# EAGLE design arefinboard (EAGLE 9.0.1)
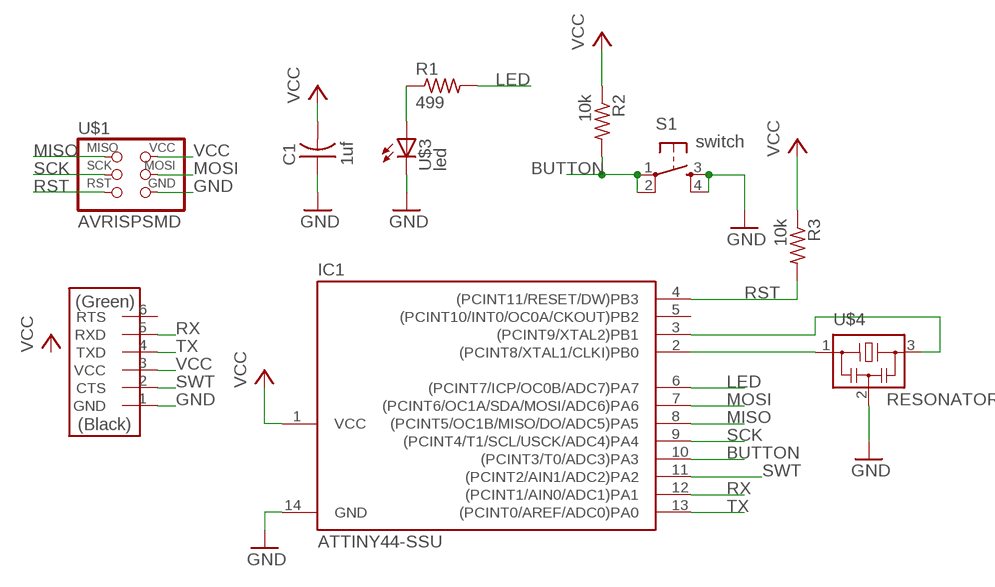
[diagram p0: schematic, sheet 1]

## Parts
C1  1uf  CAP-US1206FAB  [C1206FAB]
IC1  ATTINY44-SSU  [SOIC14]
R1  499  RES-US1206FAB  [R1206FAB]
R2  10k  RES-US1206FAB  [R1206FAB]
R3  10k  RES-US1206FAB  [R1206FAB]
S1  switch  6MM_SWITCH6MM_SWITCH  [6MM_SWITCH]
U$1  AVRISPSMD  [2X03SMD]
U$2  FTDI-SMD-HEADER  [1X06SMD]
U$3  led  LEDFAB1206  [LED1206FAB]
U$4  RESONATOR  [EFOBM]

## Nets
BUTTON: IC1.10((PCINT3/T0/ADC3)PA3) R2.2 S1.1(P) S1.2(P1)
GND: C1.1 IC1.14(GND) S1.3(S) S1.4(S1) U$1.6(GND) U$2.1(GND) U$3.2(C) U$4.2
LED: IC1.6((PCINT7/ICP/OC0B/ADC7)PA7) R1.2
MISO: IC1.8((PCINT5/OC1B/MISO/DO/ADC5)PA5) U$1.1(MISO)
MOSI: IC1.7((PCINT6/OC1A/SDA/MOSI/ADC6)PA6) U$1.4(MOSI)
N$1: R1.1 U$3.1(A)
N$10: IC1.3((PCINT9/XTAL2)PB1) U$4.3
N$11: IC1.2((PCINT8/XTAL1/CLKI)PB0) U$4.1
RST: IC1.4((PCINT11/RESET/DW)PB3) R3.2 U$1.5(RST)
RX: IC1.12((PCINT1/AIN0/ADC1)PA1) U$2.5(RXD)
SCK: IC1.9((PCINT4/T1/SCL/USCK/ADC4)PA4) U$1.3(SCK)
SWT: IC1.11((PCINT2/AIN1/ADC2)PA2) U$2.2(CTS)
TX: IC1.13((PCINT0/AREF/ADC0)PA0) U$2.4(TXD)
VCC: C1.2 IC1.1(VCC) R2.1 R3.1 U$1.2(VCC) U$2.3(VCC)
Unconnected: IC1.5((PCINT10/INT0/OC0A/CKOUT)PB2) U$2.6(RTS)

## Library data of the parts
C1 = fab:CAP-US
IC1 = fab:ATTINY44
R1-R3 = fab:RES-US: Resistor (US Symbol)
S1 = FabLab:6MM_SWITCH: OMRON SWITCH
U$1 = fab:AVRISP
U$2 = fab:FTDI-SMD-HEADER
U$3 = fab:LED: LED
U$4 = fab:RESONATOR

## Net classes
0 default: width 0.305 mm, drill 0.508 mm, clearance 0.254 mm

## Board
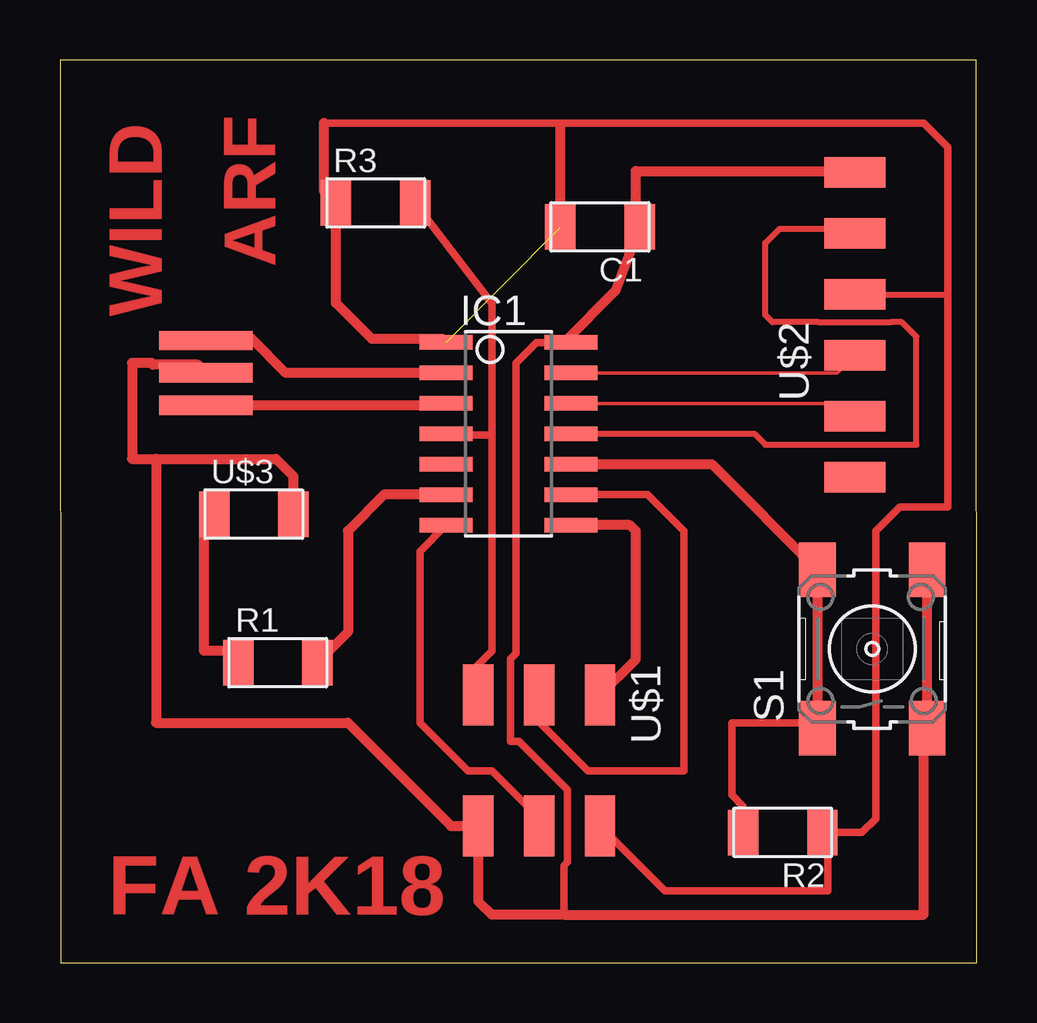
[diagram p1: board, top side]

Size 38.22 x 37.63 mm. Coordinates in mm from the lower left corner, seen from the top.
Outline: 0.03,0 38.22,0 38.19,37.63 0,37.63 0.03,0
Copper layers (1*16): Top 0.035mm / dielectric 1.5mm / Bottom 0.035mm
Design rules "default *": minimum track width 10mm, minimum drill 0.35mm, track to track 16mil, track to pad 16mil, pad to pad 16mil, via to via 16mil, smd to smd 16mil, copper to edge 40mil, drill to drill 6mil, minimum pad ring 10mil, minimum via ring 8mil, stop-mask expansion 4mil, vias tented up to drill 0mil, thermal gap 10mil

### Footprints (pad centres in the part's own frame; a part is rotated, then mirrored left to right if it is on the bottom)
C1206FAB = smd 1.27 x 1.905: 1 -1.651,0; 2 1.651,0
SOIC14 = smd 0.61 x 2.21: 1 -3.81,-2.603; 2 -2.54,-2.603; 3 -1.27,-2.603; 4 0,-2.603; 5 1.27,-2.603; 6 2.54,-2.603; 7 3.81,-2.603; 8 3.81,2.603; 9 2.54,2.603; 10 1.27,2.603; 11 0,2.603; 12 -1.27,2.603; 13 -2.54,2.603; 14 -3.81,2.603
R1206FAB = smd 1.27 x 1.905: 1 -1.651,0; 2 1.651,0
6MM_SWITCH = smd 2.286 x 1.524: 1 -3.302,2.286; 2 3.302,2.286; 3 -3.302,-2.286; 4 3.302,-2.286
2X03SMD = smd 2.54 x 1.27: 1 -2.54,2.54; 2 2.92,2.54; 3 -2.54,0; 4 2.92,0; 5 -2.54,-2.54; 6 2.92,-2.54
1X06SMD = smd 2.54 x 1.27: 1 0,6.35; 2 0,3.81; 3 0,1.27; 4 0,-1.27; 5 0,-3.81; 6 0,-6.35
LED1206FAB = smd 1.27 x 1.905: 1 -1.651,0; 2 1.651,0
EFOBM = smd 0.8 x 3.9: 1 -1.35,0; 2 0,0; 3 1.35,0

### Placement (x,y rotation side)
C1  22.51,30.67 180 top
IC1  18.7,22.05 270 top
R1  9.08,12.51 0 top
R2  30.13,5.43 180 top
R3  13.16,31.67 0 top
S1  33.86,13.08 90 top
U$1  19.97,8.62 270 top
U$2  33.13,26.59 0 top
U$3  8.08,18.7 0 top
U$4  6.08,24.59 270 top

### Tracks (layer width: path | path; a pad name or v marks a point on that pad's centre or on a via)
BUTTON
  Top 0.305: S1.1 31.35,10 28,10 28,7 28.48,6.52 R2.2
  Top 0.406: S1.1 S1.2 27.18,20.78 IC1.10 22.3,20.78
GND
  Top 0.305: IC1.14 21,25.86 19.86,25.86 19,25 19,12.88 18.78,12.66 18.78,9.22 19.14,9.22 21.16,7.2 21.16,4.2 21,4.04 21,2
  Top 0.406: S1.4 S1.3 36,9.63 36,2 21,2 18,2 17.43,2.57 U$1.6 16.3,5.7 12,10 4,10 4,21 | 4,21 9,21 9.73,20.27 U$3.2 | 21,25.86 23.16,28.02 C1.1 24,30.83 24,33 33.07,33 U$2.1 | U$4.2 5.74,24.93 3.88,24.93 3.81,25 3,25 3,21 4,21
  Top 0.508: 32.86,32.67 U$2.1
LED
  Top 0.406: IC1.6 13.51,19.51 12,18 12,13.78 R1.2
MISO
  Top 0.406: U$1.1 24,12.65 24,18 23.76,18.24 IC1.8
MOSI
  Top 0.305: 20,5.73 U$1.4 19.97,6.03 18,8 17,8 15,10 15,17.14 IC1.7
N$1
  Top 0.406: R1.1 6.94,13 6,13 6,18.27 U$3.1
N$10
  Top 0.406: U$4.3 16.02,23.24 IC1.3
N$11
  Top 0.406: IC1.2 9.41,24.59 8,26 6.14,26 U$4.1
RST
  Top 0.305: R3.2 18,27.48 18,22 | IC1.4 16.15,22 18,22 | 18,22 18,13 17,12 17,11.59 U$1.5
RX
  Top 0.152: IC1.12 32.59,23.32 U$2.5
SCK
  Top 0.305: IC1.9 24.49,19.51 26,18 26,8 22,8 20,10 20,11.13 U$1.3
SWT
  Top 0.254: 21.35,22 IC1.11 28.95,22.05 29.4,21.6 35.7,21.6 35.7,26.1 35.1,26.7 34.63,26.7 34.62,26.69 31.64,26.69 31.63,26.7 29.7,26.7 29.4,27 29.4,30 30,30.6 32.93,30.6 U$2.2
TX
  Top 0.152: IC1.13 32.4,24.59 U$2.4
VCC  (1 unrouted)
  Top 0.254: U$2.3 36.96,27.86 37,27.9
  Top 0.305: 32,5.43 33.43,5.43 34,6 34,18 35,19 37,19 37,27.9 37,34 36,35 11,35 | 32,5.43 R2.1 | U$1.2 25.21,3 32,3 32,5.43
  Top 0.406: C1.2 20.86,34.86 | IC1.1 15.96,26 13,26 11.51,27.49 R3.1 11,32.18 11,35
  Top 0.508: U$2.3 33.27,28

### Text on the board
Top: WILD | ARF | FA 2K18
